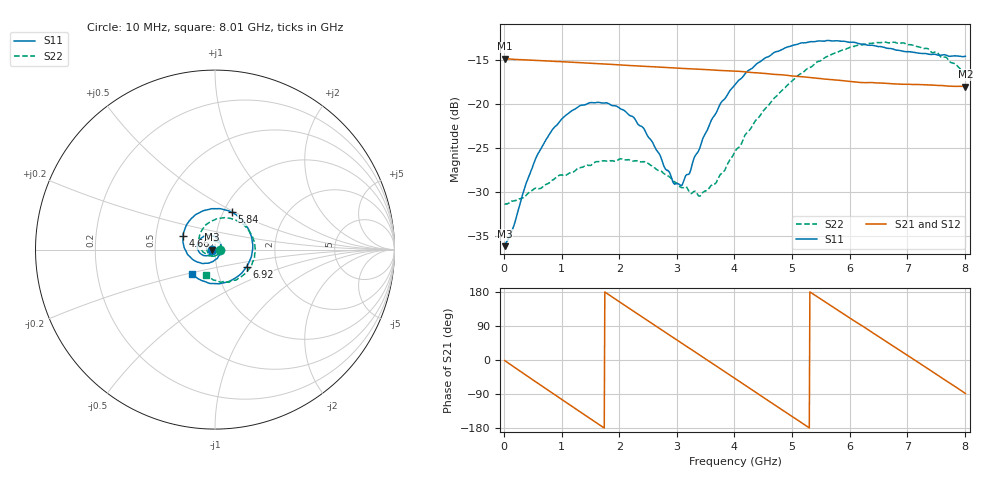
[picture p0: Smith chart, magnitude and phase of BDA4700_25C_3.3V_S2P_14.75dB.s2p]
!Agilent Technologies,E5071B,MY42404982,A.09.10
!Date: Mon Oct 20 18:09:13 2025
!Data & Calibration Information:
!Freq	S11:SOLT2(ON)	S21:SOLT2(ON)	S12:SOLT2(ON)	S22:SOLT2(ON)
# Hz S RI R 50
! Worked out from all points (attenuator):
!   801 points, 10 MHz to 8.01 GHz, reference 50 ohm
!   highest |S21| = -14.84 dB at 10 MHz (marker M1); lowest = -18.0 dB at 8.01 GHz (marker M2)
!   lowest |S11| = -36.2 dB at 10 MHz (marker M3), VSWR 1.03, Z = 48.5 - j0.117 ohm
!   |S11| at or under -10 dB: start of sweep to end of sweep
!   |S22| runs from -31.4 to -13.0 dB; largest |S21 - S12| = 0.0021
!   S11 on the Smith chart (normalised r, x): 10 MHz: 0.97, -0.00; 4.66 GHz: 0.69, +0.11; 5.84 GHz: 1.10, +0.48; 6.92 GHz: 1.39, -0.28; 8.01 GHz: 0.75, -0.21
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1e7  -0.0155 -0.00121  0.181 -0.00396  0.1809 -0.00411  0.0271 -0.000987
1.5e8  -0.0167 -0.00997  0.1726 -0.0494  0.1725 -0.0495  0.027 -0.00753
6e8  -0.0406 -0.0337  0.0811 -0.157  0.0811 -0.1569  0.0121 -0.0307
1.01e9  -0.0792 -0.0241  -0.0447 -0.1681  -0.0446 -0.1681  -0.0188 -0.0347
1.35e9  -0.0982 0.00827  -0.131 -0.1109  -0.131 -0.111  -0.0409 -0.015
1.72e9  -0.0861 0.0532  -0.1688 -0.00722  -0.1688 -0.0072  -0.0445 0.0166
2.08e9  -0.0475 0.0791  -0.1376 0.0935  -0.1377 0.0934  -0.0244 0.0415
2.42e9  -0.00104 0.073  -0.0598 0.1525  -0.0598 0.1525  0.00569 0.0466
2.68e9  0.026 0.046  0.0136 0.1616  0.0134 0.1615  0.0242 0.0342
2.94e9  0.0346 0.00833  0.0825 0.1375  0.0824 0.1372  0.0334 0.015
3.08e9  0.0316 -0.0135  0.1133 0.1122  0.1122 0.113  0.0334 0.00194
3.41e9  -0.0006 -0.0577  0.1542 0.0322  0.1543 0.0321  0.0183 -0.0239
3.67e9  -0.0441 -0.0758  0.1508 -0.0389  0.1509 -0.0392  -0.0049 -0.035
4.01e9  -0.1128 -0.0619  0.1012 -0.1158  0.1014 -0.1154  -0.0444 -0.0299
4.66e9  -0.1778 0.0752  -0.0617 -0.1341  -0.0613 -0.1346  -0.0896 0.0554
5.35e9  -0.0576 0.2185  -0.1407 0.0104  -0.1407 0.00951  -0.00685 0.1636
5.84e9  0.0934 0.2076  -0.082 0.1087  -0.0816 0.1087  0.1145 0.1648
6.26e9  0.1874 0.1122  0.00886 0.132  0.0108 0.1315  0.1994 0.0883
6.68e9  0.2055 -0.0236  0.0935 0.0913  0.0938 0.0911  0.2214 -0.0244
6.92e9  0.1755 -0.0954  0.1212 0.046  0.1212 0.0453  0.2034 -0.0908
7.47e9  0.0277 -0.1898  0.1059 -0.0717  0.1058 -0.0719  0.0814 -0.1793
8.01e9  -0.1282 -0.1358  0.00359 -0.1257  0.00405 -0.1258  -0.0479 -0.1421
